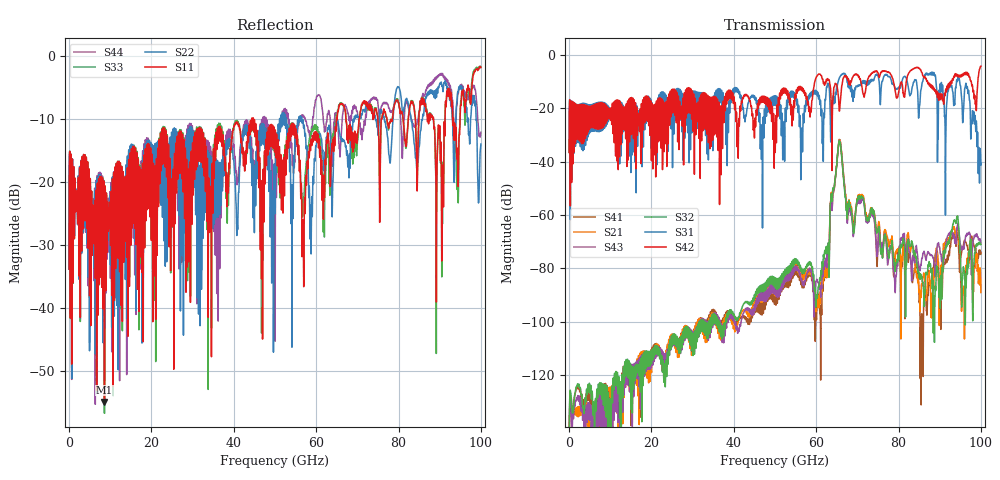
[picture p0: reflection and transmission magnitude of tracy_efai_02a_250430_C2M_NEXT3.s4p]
!! PART DESCRIPTION: TE 224G+ VSR Channel- Chip to module, IO connector to CPC(Co-packaged connector) through over the board cable
!! CHANNEL DESCRIPTION: Module trace -> Mated IO 224G+ Connector -> Internal Cable Termination -> 30AWG 300mm Cable -> Cable
!!  termination + CPC connector(No footprint or package included)
!! MODEL REVISION:  Rev 3, Created on April 29, 2025
!! MODEL STATUS: Development
!! MODEL GEOMETRY: NEXT3
!! MODEL FREQUENCY RANGE: 0 GHz to 100 GHz in 10.00 MHz frequency steps
!! PORT DEFINITIONS:
!! Port  1  ----->  Module Side  -->  Module Side  <-----  Port  2
!! Port  3  ----->  Module Side  -->  Module Side  <-----  Port  4
# HZ S MA R 45.000000
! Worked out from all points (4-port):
!   10000 points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, 10 MHz to 100 GHz, reference 45 ohm
!   strongest paths, dB at 10 MHz, 25.01 GHz, 50.01 GHz, 75.01 GHz, 100 GHz:
!     S42: -36.5, -16.7, -29.8, -6.7, -4.3
!     S31: -36.5, -17.8, -16.0, -7.7, -40.6
!     S32: -144.0, -109.0, -84.0, -65.8, -71.0
!     S43: -146.5, -109.3, -86.1, -70.9, -70.4
!     S21: -147.7, -108.4, -86.0, -64.8, -89.0
!     S41: -144.4, -108.3, -88.6, -70.5, -74.0
!   lowest |S11| = -54.9 dB at 8.6 GHz (marker M1), VSWR 1.00, Z = 44.9 + j0.15 ohm
!   |S11| at or under -10 dB: start of sweep to 44.32 GHz; 44.72 GHz to 64.9 GHz (20.18 GHz wide, 36.8 % of centre); 67.23 GHz to 70.41 GHz (3.185 GHz wide, 4.63 % of centre)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
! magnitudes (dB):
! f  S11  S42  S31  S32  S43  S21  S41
! 10 MHz  -33.8  -36.5  -36.5  -144.0  -146.5  -147.7  -144.4
! 8.6 GHz  -54.9  -25.2  -27.5  -126.2  -132.4  -128.3  -126.1
! 62.12 GHz  -18.0  -10.7  -17.7  -73.7  -77.6  -79.8  -81.0
! 65.69 GHz  -7.8  -20.6  -8.3  -32.6  -32.3  -32.2  -31.9
! 79.14 GHz  -7.4  -13.2  -12.4  -81.1  -87.5  -77.2  -76.3
! 94.55 GHz  -18.1  -8.1  -9.1  -63.1  -64.6  -66.9  -71.1
! 100 GHz  -1.8  -4.3  -40.6  -71.0  -70.4  -89.0  -74.0
